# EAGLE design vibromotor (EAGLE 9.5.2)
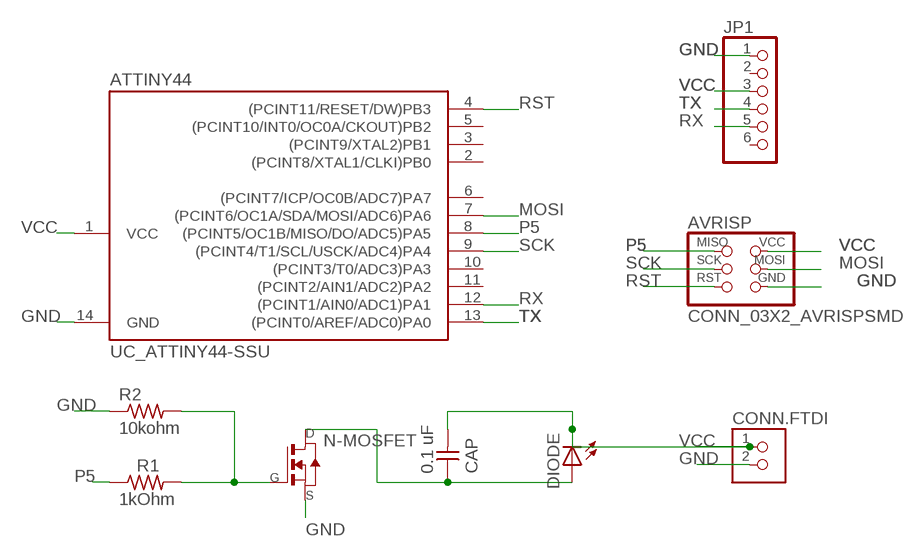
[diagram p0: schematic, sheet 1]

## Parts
ATTINY44  UC_ATTINY44-SSU  [SOIC14]
AVRISP  CONN_03X2_AVRISPSMD  [2X03SMD]
CAP  0.1 uF  CAP_UNPOLARIZEDFAB  [C1206FAB]
CONN.FTDI  CONN_02_TERM-FABLAB  [ED555DS-2DS]
DIODE  LEDFAB1206  [LED1206FAB]
JP1  PINHD-1X6  [1X06]
N-MOSFET  MOSFET_NSOT23  [SOT-23]
R1  1kOhm  R1206FAB  [R1206FAB]
R2  10kohm  R1206FAB  [R1206FAB]

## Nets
GND: ATTINY44.14(GND) AVRISP.6(GND) CONN.FTDI.2 JP1.1 N-MOSFET.2(S) R2.1
MOSI: ATTINY44.7((PCINT6/OC1A/SDA/MOSI/ADC6)PA6) AVRISP.4(MOSI)
N$1: N-MOSFET.3(G) R1.2 R2.2
N$2: CAP.1 DIODE.1(A) N-MOSFET.1(D)
P5: ATTINY44.8((PCINT5/OC1B/MISO/DO/ADC5)PA5) AVRISP.1(MISO) R1.1
RST: ATTINY44.4((PCINT11/RESET/DW)PB3) AVRISP.5(RST)
RX: ATTINY44.12((PCINT1/AIN0/ADC1)PA1) JP1.5
SCK: ATTINY44.9((PCINT4/T1/SCL/USCK/ADC4)PA4) AVRISP.3(SCK)
TX: ATTINY44.13((PCINT0/AREF/ADC0)PA0) JP1.4
VCC: ATTINY44.1(VCC) AVRISP.2(VCC) CAP.2 CONN.FTDI.1 DIODE.2(C) JP1.3
Unconnected: ATTINY44.2((PCINT8/XTAL1/CLKI)PB0) ATTINY44.3((PCINT9/XTAL2)PB1) ATTINY44.5((PCINT10/INT0/OC0A/CKOUT)PB2) ATTINY44.6((PCINT7/ICP/OC0B/ADC7)PA7) ATTINY44.10((PCINT3/T0/ADC3)PA3) ATTINY44.11((PCINT2/AIN1/ADC2)PA2) JP1.2 JP1.6

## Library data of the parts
ATTINY44 = fab:UC_ATTINY44
AVRISP = fab:CONN_03X2_AVRISP
CAP = fab:CAP_UNPOLARIZED
CONN.FTDI = fab:CONN_02_TERM: 3.5mm terminal block, 2 positions ED555-2DS as found in the fablab inventory.
DIODE = fab:LED: LED
JP1 = pinhead:PINHD-1X6: PIN HEADER
N-MOSFET = fab:MOSFET_N: MOS FET
R1 R2 = fab:R: Resistor (US Symbol)

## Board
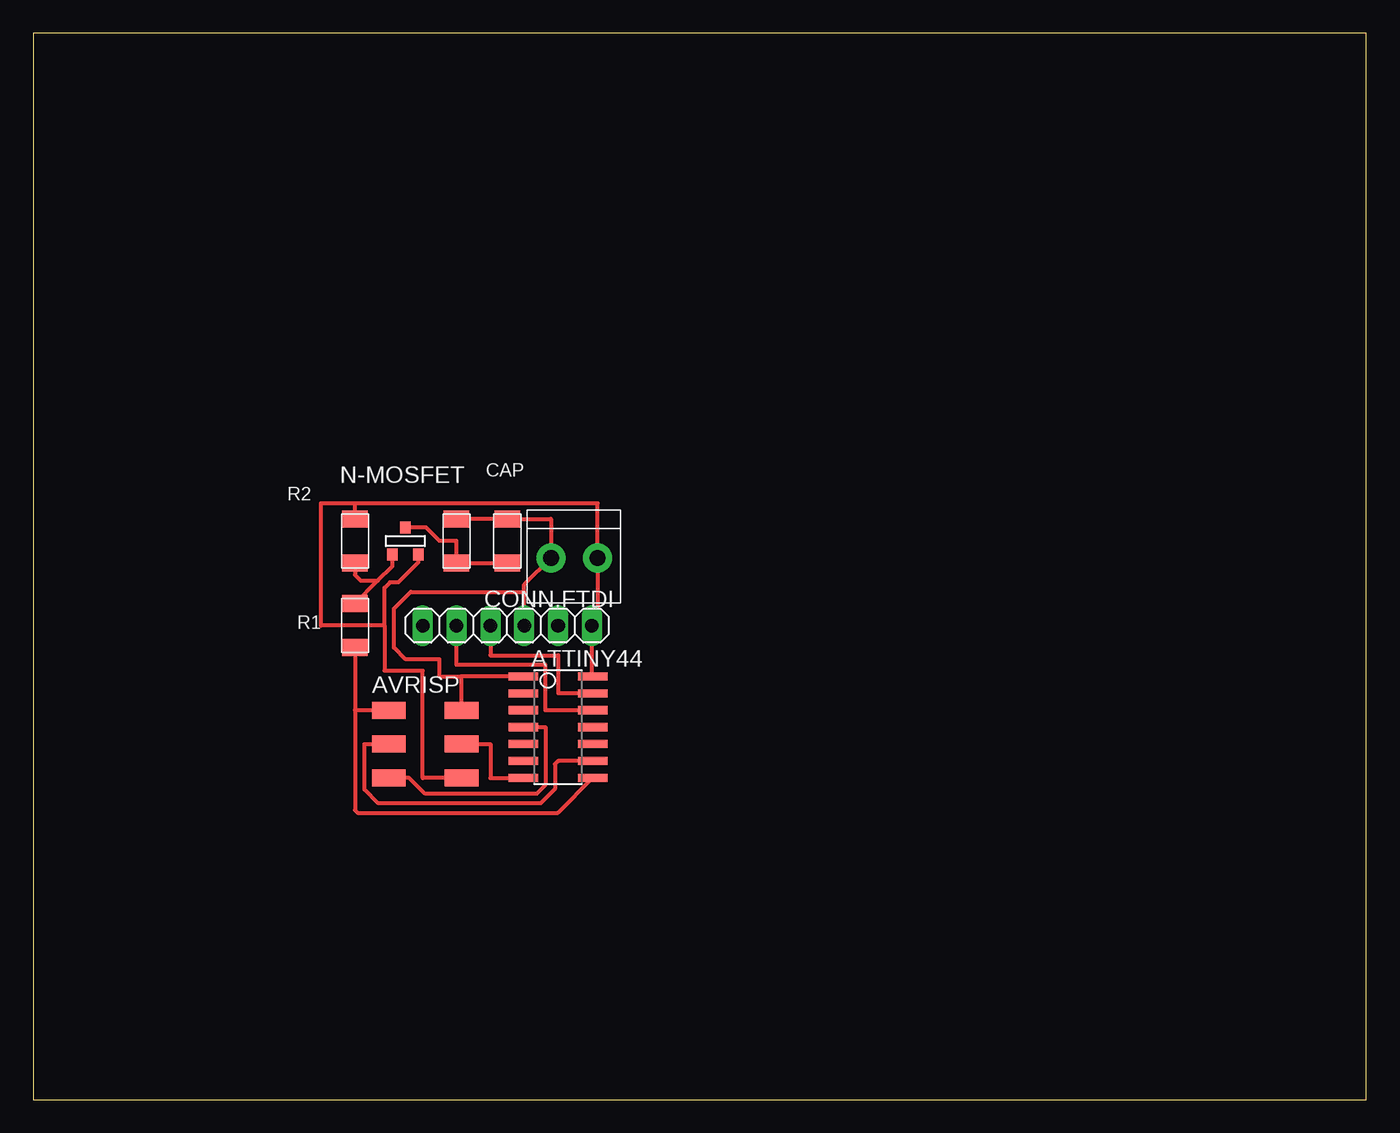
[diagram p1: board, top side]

Size 100 x 80 mm. Coordinates in mm from the lower left corner, seen from the top.
Outline: 0,0 100,0 100,80 0,80 0,0
Copper layers (1*16): Top 0.035mm / dielectric 1.5mm / Bottom 0.035mm
Design rules "default *": minimum track width 12mil, minimum drill 32mil, track to track 16mil, track to pad 16mil, pad to pad 16mil, via to via 16mil, smd to smd 16mil, copper to edge 16mil, drill to drill 16mil, minimum pad ring 10mil, minimum via ring 8mil, stop-mask expansion 4mil, vias tented up to drill 0mil, thermal gap 10mil

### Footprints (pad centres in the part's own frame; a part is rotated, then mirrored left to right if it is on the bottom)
SOIC14 = smd 0.61 x 2.21: 1 -3.81,-2.603; 2 -2.54,-2.603; 3 -1.27,-2.603; 4 0,-2.603; 5 1.27,-2.603; 6 2.54,-2.603; 7 3.81,-2.603; 8 3.81,2.603; 9 2.54,2.603; 10 1.27,2.603; 11 0,2.603; 12 -1.27,2.603; 13 -2.54,2.603; 14 -3.81,2.603
2X03SMD = smd 2.54 x 1.27: 1 -2.54,2.54; 2 2.92,2.54; 3 -2.54,0; 4 2.92,0; 5 -2.54,-2.54; 6 2.92,-2.54
C1206FAB = smd 1.27 x 1.905: 1 -1.651,0; 2 1.651,0
ED555DS-2DS = drill 1.2 pad 2.184: 1 1.8,0; 2 -1.7,0
LED1206FAB = smd 1.27 x 1.905: 1 -1.651,0; 2 1.651,0
1X06 = drill 1.016 long: 1 -6.35,0; 2 -3.81,0; 3 -1.27,0; 4 1.27,0; 5 3.81,0; 6 6.35,0
SOT-23 = smd 0.787 x 0.889: 1 0.025,-1.016; 2 -0.94,1.016; 3 0.991,1.016
R1206FAB = smd 1.27 x 1.905: 1 -1.651,0; 2 1.651,0

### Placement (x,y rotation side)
ATTINY44  39.37,27.94 270 top
AVRISP  29.21,26.67 0 top
CAP  31.75,41.91 90 top
CONN.FTDI  40.64,40.64 180 top
DIODE  35.56,41.91 90 top
JP1  35.56,35.56 180 top
N-MOSFET  27.94,41.91 180 top
R1  24.13,35.56 90 top
R2  24.13,41.91 270 top

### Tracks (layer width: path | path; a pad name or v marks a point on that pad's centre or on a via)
GND
  Top 0.305: ATTINY44.14 41.91,31.75 JP1.1 42.34,35.99 CONN.FTDI.2 42.34,44.76 24.13,44.76 | AVRISP.6 29.21,24.13 29.21,32.16 26.34,32.16 26.34,35.56 | 24.13,44.76 21.59,44.76 21.59,35.56 26.34,35.56 | 26.34,35.56 26.34,38.4 26.76,38.81 27.38,38.81 28.88,40.31 N-MOSFET.2 | R2.1 24.13,44.76
MOSI
  Top 0.305: AVRISP.4 34.29,26.67 34.29,24.13 ATTINY44.7
N$1
  Top 0.305: R1.2 25.84,38.92 | 25.84,38.92 26.95,40.03 N-MOSFET.3 | R2.2 24.13,39.37 24.57,38.92 25.84,38.92
N$2
  Top 0.305: DIODE.1 CAP.1 31.75,41.91 30.48,41.91 29.46,42.93 N-MOSFET.1
P5
  Top 0.305: ATTINY44.8 39.36,21.51 24.32,21.51 24.13,21.7 24.13,29.21 | AVRISP.1 24.13,29.21 | R1.1 24.13,29.21
RST
  Top 0.305: AVRISP.5 28.2,24.13 29.4,22.94 37.77,22.94 38.43,23.59 38.43,27.94 ATTINY44.4
RX
  Top 0.305: ATTINY44.12 38.43,29.21 38.43,32.61 31.75,32.61 JP1.5
SCK
  Top 0.305: ATTINY44.9 39.37,25.4 39.14,25.17 39.14,23.3 38.07,22.23 25.88,22.23 24.84,23.26 24.84,26.67 AVRISP.3
TX
  Top 0.305: ATTINY44.13 39.37,30.48 39.37,33.33 34.29,33.33 JP1.4
VCC
  Top 0.305: CAP.2 DIODE.2 38.84,43.56 CONN.FTDI.1 36.83,38.63 36.83,38.1 | JP1.3 36.83,38.1 | ATTINY44.1 32.13,31.75 | 32.13,31.75 30.48,31.75 30.48,33.02 27.94,33.02 27.05,33.91 27.05,36.83 28.32,38.1 36.83,38.1 | AVRISP.2 32.13,31.75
